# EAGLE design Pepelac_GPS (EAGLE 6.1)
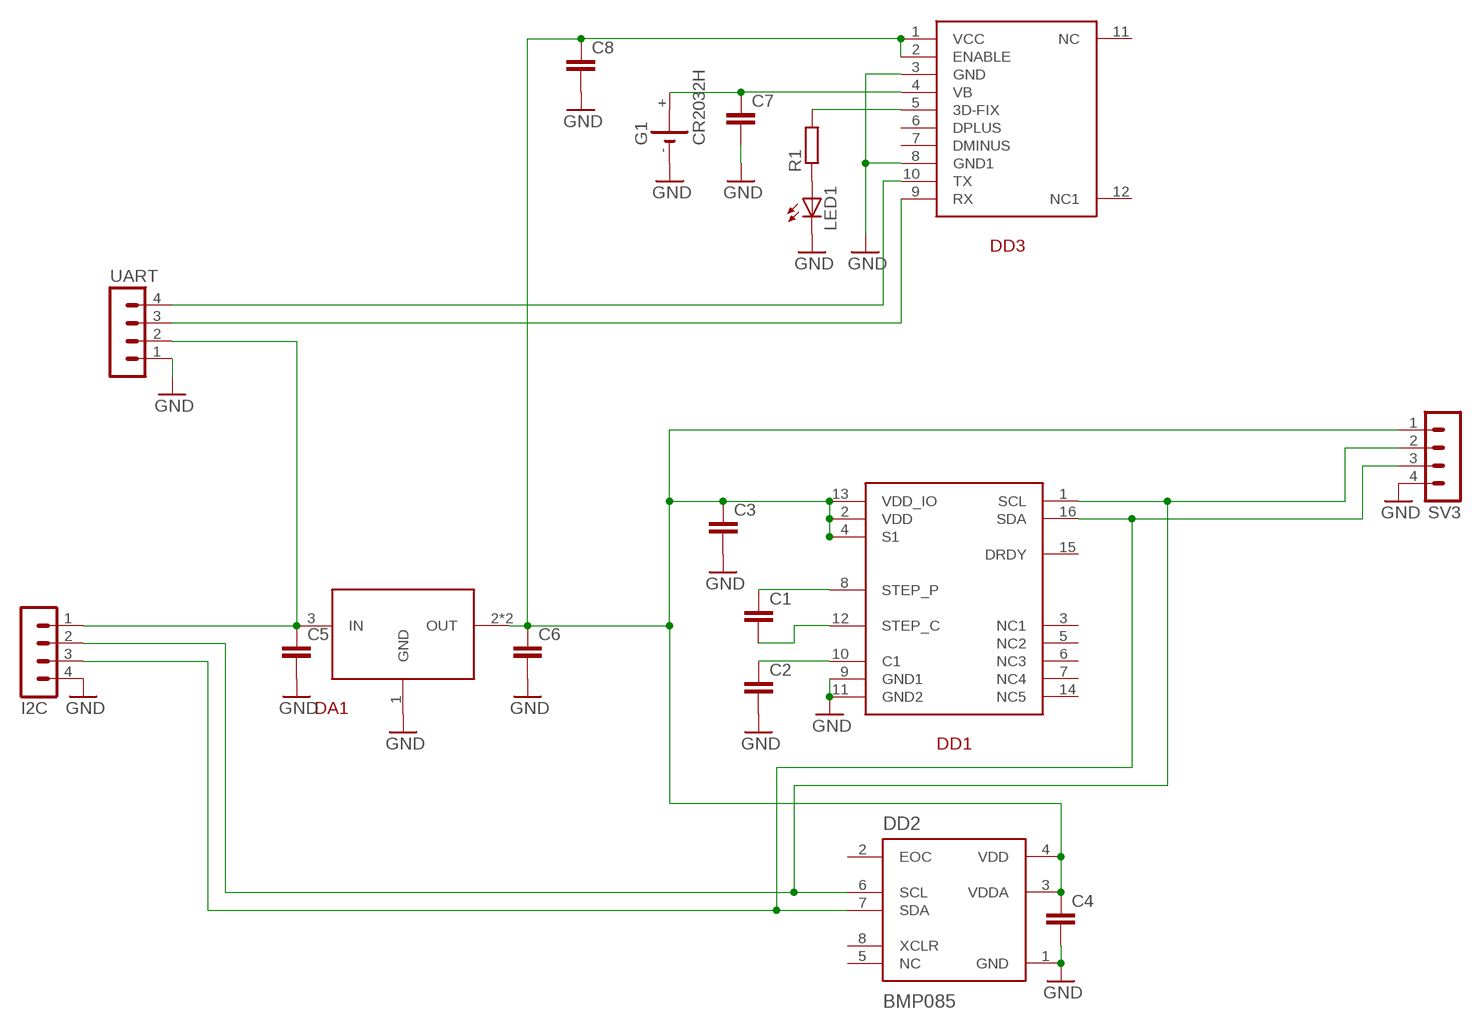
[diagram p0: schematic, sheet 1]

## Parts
C1  C-EUC3216  [C3216]
C2  C-EUC3216  [C3216]
C3  C-EUC3216  [C3216]
C4  C-EUC3216  [C3216]
C5  C-EUC3216  [C3216]
C6  C-EUC3216  [C3216]
C7  C-EUC3216  [C3216]
C8  C-EUC3216  [C3216]
DA1  1117  [SOT223-W]
DD1  HMC5883L  [LCC-16]
DD2  BMP085  [QFN127P500X500X120-8N]
DD3  FGPMMOPA6B  [FGPMMOPA6B]
G1  CR2032H  [CR2032H]
I2C  MA04-1  [MA04-1]
LED1  LEDKA-3528ASYC  [KA-3528ASYC]
R1  R-EU_M3216  [M3216]
SV3  MA04-1  [MA04-1]
UART  MA04-1  [MA04-1]

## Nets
GND: C2.2 C3.2 C4.2 C5.2 C6.2 C7.2 C8.2 DA1.1(GND) DD1.9(GND1) DD1.11(GND2) DD2.1(GND) DD3.3(GND) DD3.8(GND1) G1.- I2C.4 LED1.C SV3.4 UART.1
N$2: C5.1 DA1.3(IN) I2C.1 UART.2
N$3: C3.1 C4.1 C6.1 C8.1 DA1.2(OUT) DA1.4(OUT) DD1.2(VDD) DD1.4(S1) DD1.13(VDD_IO) DD2.3(VDDA) DD2.4(VDD) DD3.1(VCC) DD3.2(ENABLE) SV3.1
N$4: LED1.A R1.1
N$5: DD1.16(SDA) DD2.7(SDA) I2C.3 SV3.3
N$6: DD1.1(SCL) DD2.6(SCL) I2C.2 SV3.2
N$8: C7.1 DD3.4(VB) G1.+
N$11: DD3.5(3D-FIX) R1.2
N$15: DD3.10(TX) UART.4
N$16: DD3.9(RX) UART.3
N$17: C1.1 DD1.8(STEP_P)
N$18: C1.2 DD1.12(STEP_C)
N$19: C2.1 DD1.10(C1)
Unconnected: DD1.3(NC1) DD1.5(NC2) DD1.6(NC3) DD1.7(NC4) DD1.14(NC5) DD1.15(DRDY) DD2.2(EOC) DD2.5(NC) DD2.8(XCLR) DD3.6(DPLUS) DD3.7(DMINUS) DD3.11(NC) DD3.12(NC1) G1.+@1(+)

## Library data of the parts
C1-C8 = resistor:C-EU: CAPACITOR, European symbol
DA1 = pepelac:1117
DD1 = pepelac:HMC5883L
DD2 = pepelac:BMP085: BMP085 Digital pressure sensor
DD3 = pepelac:FGPMMOPA6B
G1 = battery:CR2032H: LI BATTERY Varta
I2C SV3 UART = con-lstb:MA04-1: PIN HEADER; OC_FARNELL: unknown; OC_NEWARK: unknown
LED1 = led:LED: LED
R1 = resistor:R-EU_: RESISTOR, European symbol

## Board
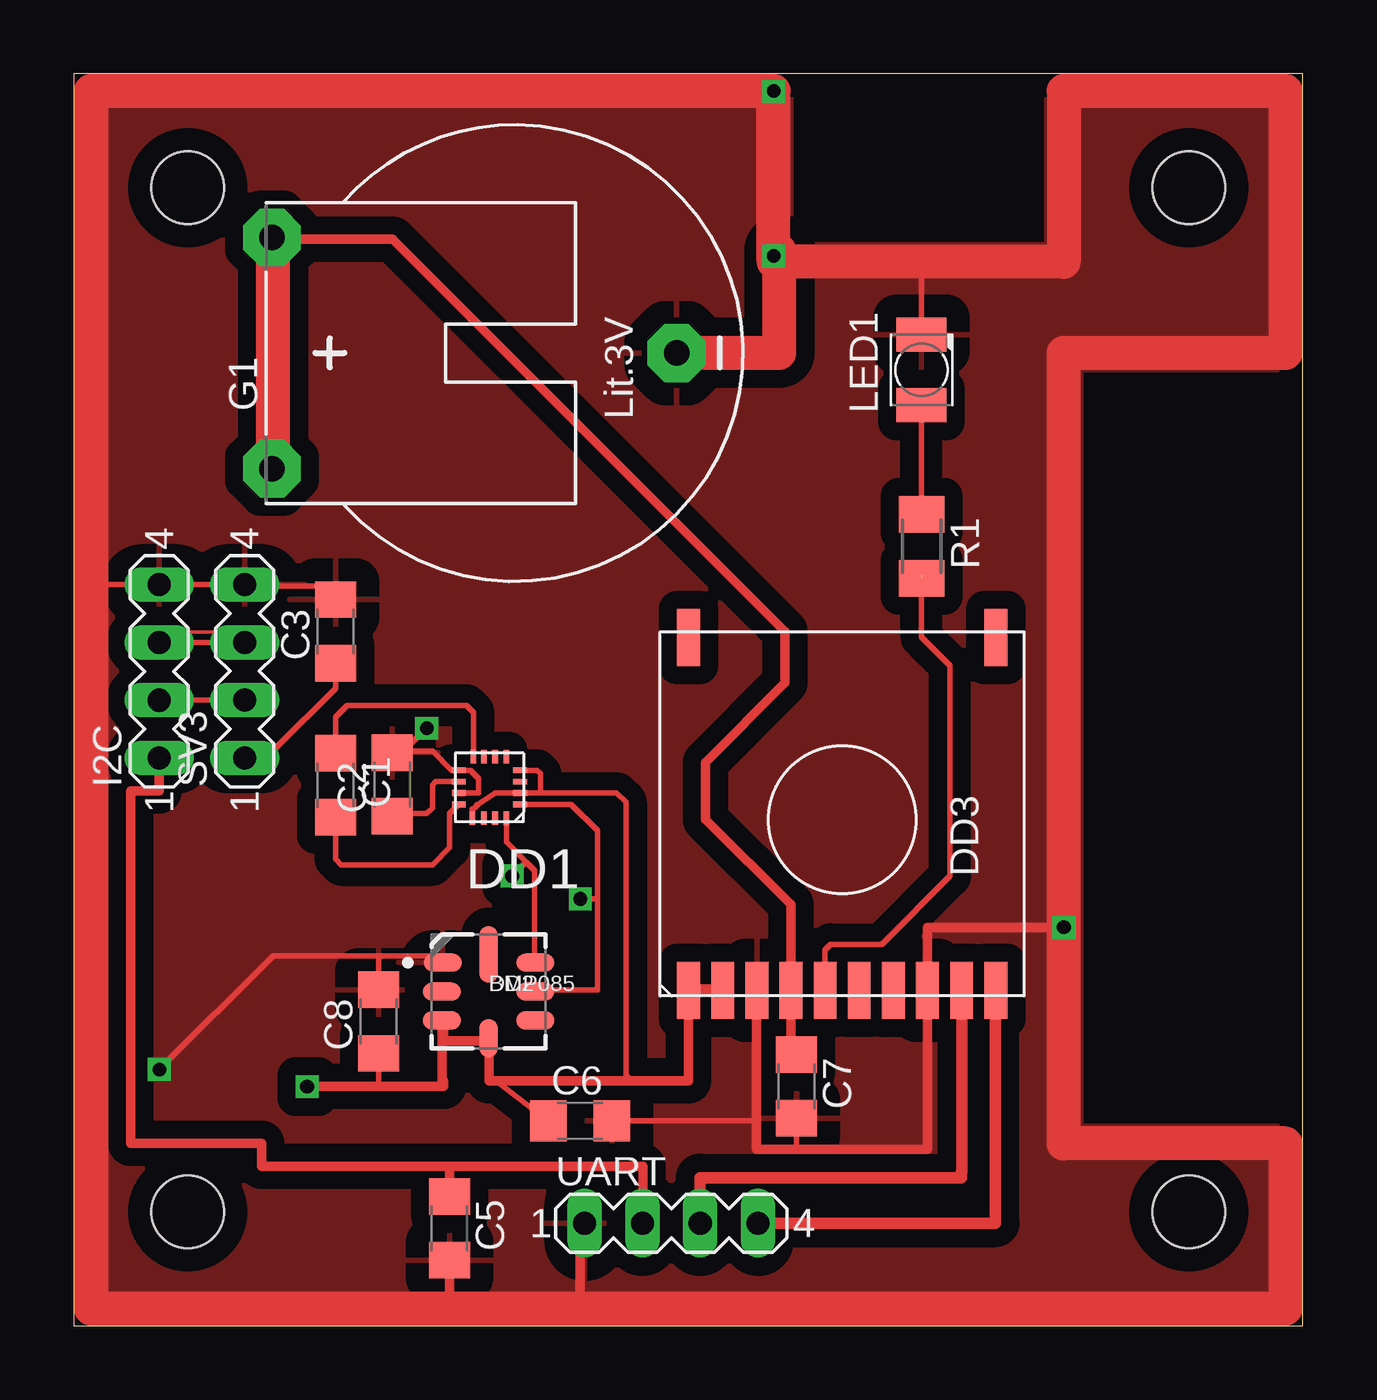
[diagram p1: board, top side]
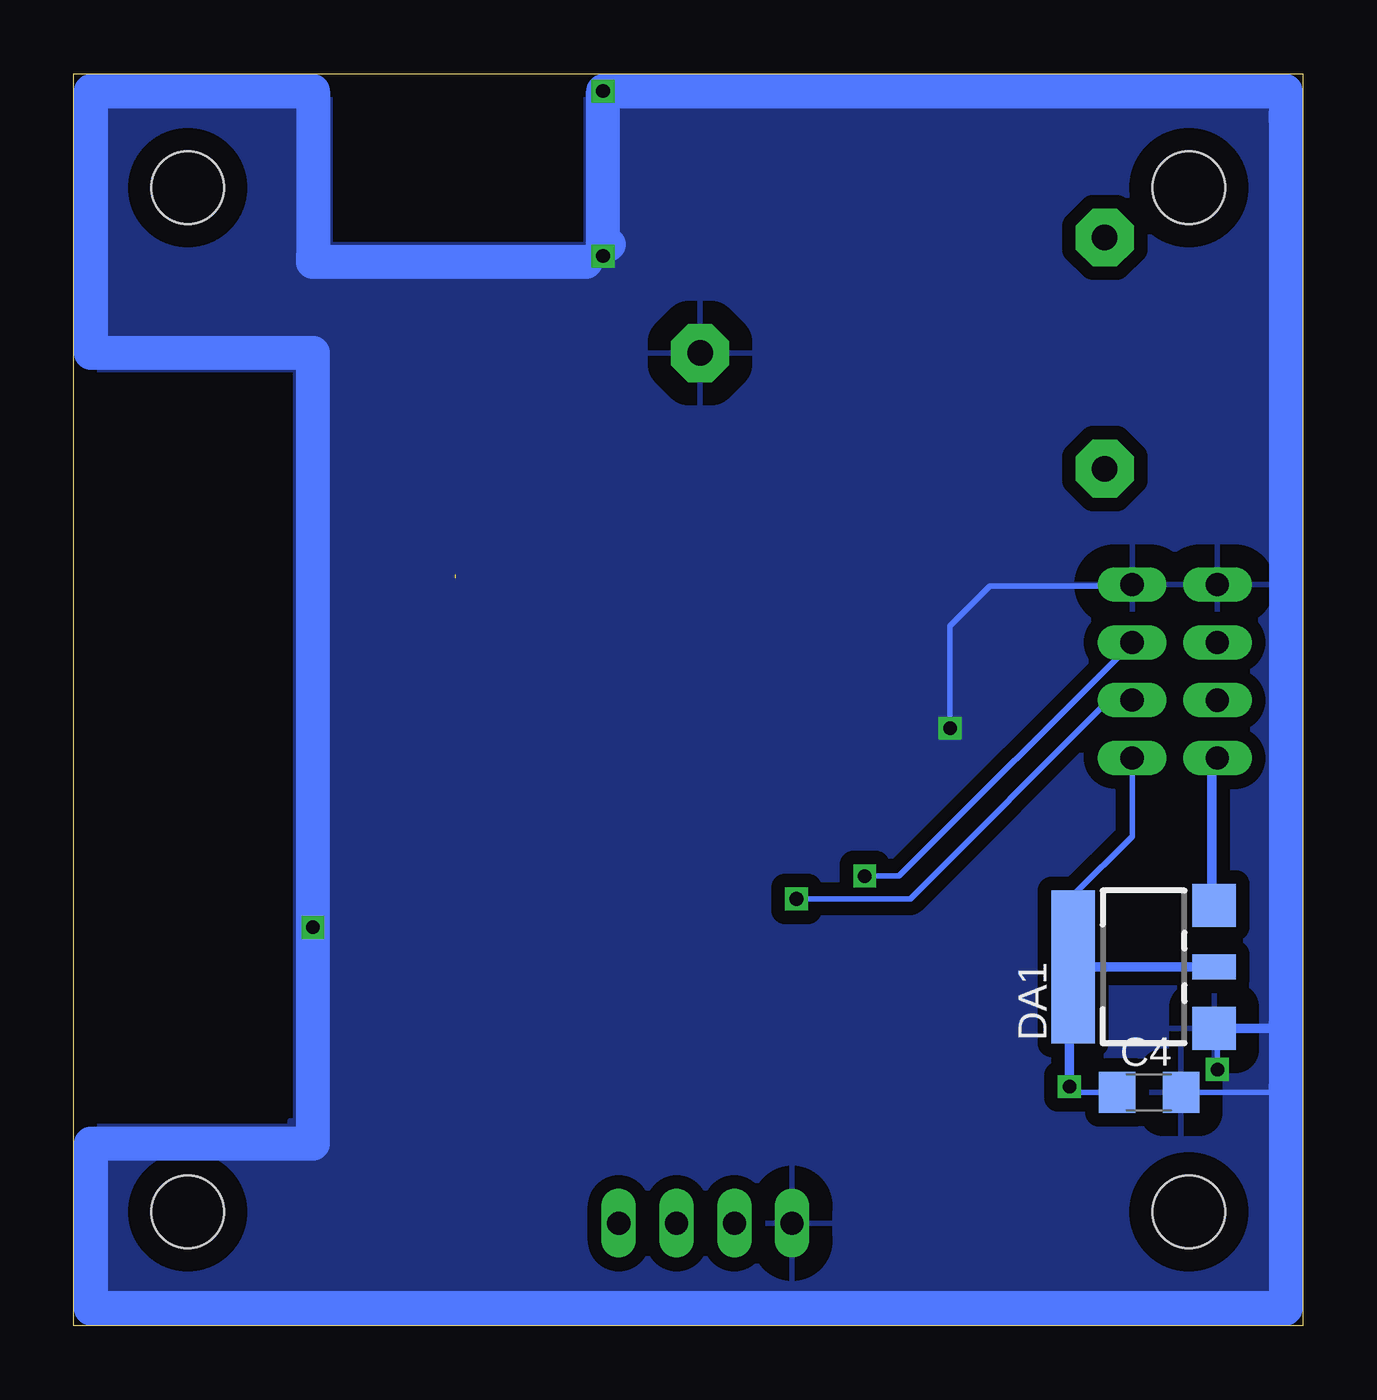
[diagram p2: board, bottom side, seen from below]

Size 54 x 55 mm. Coordinates in mm from the lower left corner, seen from the top.
Outline: 0,0 54,0 54,55 0,55 0,0
Copper layers (1*16): Top 0.035mm / dielectric 1.5mm / Bottom 0.035mm
Design rules: minimum track width 6mil, minimum drill 30mil, track to track 6mil, track to pad 6mil, pad to pad 8mil, via to via 8mil, smd to smd 8mil, copper to edge 40mil, drill to drill 8mil, minimum pad ring 10mil, minimum via ring 8mil, stop-mask expansion 4mil, vias tented up to drill 0mil, thermal gap 40mil
Holes 3.2 mm at 5,50 49,50 49,5 5,5

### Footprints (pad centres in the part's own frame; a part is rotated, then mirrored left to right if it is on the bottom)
C3216 = smd 1.6 x 1.8: 1 -1.4,0; 2 1.4,0
SOT223-W = smd 1.9 x 1.9: 1 -2.7,-3.1; 3 2.7,-3.1 | smd 1.1 x 1.9: 2 0,-3.1 | smd 6.7 x 1.9: 4 0,3.1
LCC-16 = smd 0.6 x 0.25: 1 -1.35,0.85; 2 -1.35,0.35; 3 -1.35,-0.15; 4 -1.35,-0.65; 9 1.35,-0.65; 10 1.35,-0.15; 11 1.35,0.35; 12 1.35,0.85 | smd 0.25 x 0.6: 5 -0.75,-1.25; 6 -0.25,-1.25; 7 0.25,-1.25; 8 0.7,-1.25; 13 0.75,1.45; 14 0.25,1.45; 15 -0.25,1.45; 16 -0.75,1.45
QFN127P500X500X120-8N = smd 1.67 x 0.8: 1 -2.01,1.27; 2 -2.05,0; 3 -2.05,-1.27; 5 2.05,-1.27; 6 2.05,0; 7 2.05,1.27 | smd 0.8 x 1.67: 4 0,-2.05 | smd 0.8 x 2.5: 8 0,1.63
FGPMMOPA6B = smd 2.5 x 1: 1 -7.5,6.75; 2 -7.5,5.25; 3 -7.5,3.75; 4 -7.5,2.25; 5 -7.5,0.75; 6 -7.5,-0.75; 7 -7.5,-2.25; 8 -7.5,-3.75; 9 -7.5,-5.25; 10 -7.5,-6.75; 11 8,6.75; 12 8,-6.75
CR2032H = drill 1.118 pad 2.54 octagon: + 5.08,10.795; +@1 -5.08,10.795; - 0,-6.985
MA04-1 = drill 1.016 long: 1 -3.81,0; 2 -1.27,0; 3 1.27,0; 4 3.81,0
KA-3528ASYC = smd 1.5 x 2.2: A -1.55,0; C 1.55,0
M3216 = smd 1.6 x 2: 1 -1.4,0; 2 1.4,0

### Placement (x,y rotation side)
C1  11.49,23.74 270 top
C2  13.99,23.78 90 top
C3  11.5,30.51 90 top
C4  6.76,10.25 0 bottom
C5  16.5,4.27 270 top
C6  22.24,9 0 top
C7  31.75,10.51 270 top
C8  13.39,13.36 90 top
DA1  7,15.76 90 bottom
DD1  18.26,23.75 180 top
DD2  18.22,14.68 0 top
DD3  33.76,22.23 90 top
G1  19.5,42.73 90 top
I2C  3.75,28.75 90 top
LED1  37.25,41.99 90 top
R1  37.25,34.24 270 top
SV3  7.5,28.75 90 top
UART  26.25,4.5 0 top

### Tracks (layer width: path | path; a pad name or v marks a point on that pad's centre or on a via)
GND  (via drill 0.6)
  Top 0.25: SV3.4 I2C.4 | SV3.4 0.94,32.56 0.75,32.75 | G1.- 30.48,42.73 31.25,43.5 31.25,46.5 v30.75,47 | DD1.11 17.79,23.4 17.79,24.03 17.46,24.36 17.46,24.37 17.43,24.4 DD1.9 16.6,24.4 15.75,25.25 14.06,25.25 C2.2 14.43,25.18 v15.5,26.25 | C3.2 11.35,31.91 10.75,32.5 7.56,32.5 SV3.4 | C6.2 30,9 | 30,9 | C7.2 31.75,7.75 | LED1.C 37.25,46.75 | C8.2 13.39,16.14 13.5,16.25 | 13.5,16.25 15.91,16.25 DD2.1 | 13.5,16.25 8.75,16.25 v3.75,11.25
  Top 0.406: DD3.3 30,9 30,7.75 31.75,7.75 37.5,7.75 37.5,14.75 | DD3.8 37.5,17.5 v43.5,17.5 | 22.46,4.5 22.25,4.5 22.25,0.75 | C5.2 16.5,1 16.75,0.75
  Top 0.5: UART.1 22.46,4.5 | DD3.3 | DD3.8
  Top 1.5: 0.75,54.25 0.75,32.75 0.75,0.75 16.75,0.75 22.25,0.75 53.25,0.75 53.25,8 43.5,8 v43.5,17.5 43.5,42.75 53.25,42.75 53.25,54.25 43.5,54.25 43.5,46.75 37.25,46.75 30.75,46.75 v30.75,47 v30.75,54.25 0.75,54.25
  Bottom 0.25: C4.2 1,10.25 0.75,10.5 | v15.5,26.25 15.5,30.75 13.75,32.5 7.56,32.5 SV3.4 | v3.75,11.25 3.75,12.91 DA1.1
  Bottom 0.406: DA1.1 0.94,13.06 0.75,13.25
  Bottom 0.5: 43.5,47 31.5,47 31.5,46.75
  Bottom 1.5: 31.5,46.75 43.5,46.75 43.5,47 43.5,54.25 53.25,54.25 53.25,42.75 43.5,42.75 v43.5,17.5 43.5,8 53.25,8 53.25,0.75 0.75,0.75 0.75,10.5 0.75,13.25 0.75,53 | 30.5,47.5 30.75,47.5 v30.75,54.25 0.75,54.25 0.75,53.25
  pour Bottom (isolate 0.6): 0,0 54,0 54,8.75 44.5,8.75 44.5,9 44.25,9 44.25,42 54,42 54,55 42.75,55 42.75,47.5 31.5,47.5 31.5,55 0,55
  pour Top (isolate 0.8): 0,55 31.5,55 31.5,47.5 42.75,47.5 42.75,47.75 42.75,55 54,55 54,42 44.25,42 44.25,8.75 54,8.75 54,0 0,0
N$1
  Top 1.5: 26.5,42.75 31,42.75 31,47.25
N$2
  Top 0.406: UART.2 25,4.5 25,7 16.5,7 | 16.5,7 8.25,7 8.25,8 2.5,8 2.5,23.5 3.75,23.5 I2C.1 | C5.1 16.5,7
  Bottom 0.406: I2C.1 4,24.94 4,18.5 3.9,18.5 DA1.3
N$3  (via drill 0.6)
  Top 0.152: 8.89,25.39 8.89,25.4 7.62,25.4 SV3.1
  Top 0.25: 20.5,23.4 DD1.2 19.51,23.4 19.5,23.41 | 20.5,23.4 23.85,23.4 24.25,23 24.25,11 24.5,10.75 | C6.1 18.66,10.66 18.75,10.75 | C3.1 11.5,28 8.89,25.39 8.75,25.25 7.75,25.25 7.5,25 | DD1.13 17.51,22.71 17.55,22.71 17.69,22.85 | 17.69,22.85 | 17.69,22.85 17.73,22.89 17.63,22.77 17.75,22.89 18.5,23.4 18.52,23.41 19.5,23.41 | 19.5,23.41 19.6,23.41 DD1.2 | DD1.4 20.35,24.4 20.5,24.25 20.5,23.4 | C8.1 13.39,10.61 13.5,10.5
  Top 0.406: v10.25,10.5 13.5,10.5 16.25,10.5 16.25,10.75 16.17,10.75 DD2.3 16.25,13.41 16.25,12.5 18.22,12.5 DD2.4 18.25,12.63 18.25,10.75 18.75,10.75 24.5,10.75 27,10.75 27,11 27.01,11 DD3.1
  Top 0.5: 27.01,15 DD3.1 27,14.75 28.51,14.75 DD3.2
  Bottom 0.25: DA1.4 10.1,18.91 7.5,21.5 SV3.1 | SV3.1 | C4.1 10,10.25 v10.25,10.5
  Bottom 0.406: DA1.2 DA1.4 10.25,15.76 v10.25,10.5
N$4
  Top 0.25: R1.1 LED1.A
N$5  (via drill 0.6)
  Top 0.152: I2C.3 3.81,30.48 6.35,30.48 SV3.3
  Top 0.25: DD1.16 19.01,21.24 19.88,20.38 | 19.88,20.38 20.25,20 20.25,15.97 DD2.7 | v19.25,19.75 19.88,20.38 | SV3.3 3.77,30.02 3.75,30
  Bottom 0.25: SV3.3 7.5,30 17.75,19.75 v19.25,19.75
N$6  (via drill 0.6)
  Top 0.25: DD1.1 21.85,22.9 23,21.75 23,18.75 | 23,18.75 23,14.75 20.34,14.75 DD2.6 | v22.25,18.75 23,18.75 | SV3.2 I2C.2
  Bottom 0.25: SV3.2 8.52,27.48 17.25,18.75 v22.25,18.75
N$8
  Top 0.406: C7.1 31.5,11.91 DD3.4 31.5,18.5 27.75,22.25 27.75,24.75 31.25,28.25 31.25,30.5 14,47.75 9.25,47.75 8.77,47.75 G1.+
  Top 0.5: DD3.4
  Top 1.5: 8.75,38 8.75,47.75 9.25,47.75
N$11  (1 unrouted)
  Top 0.152: 36.83,33.02 R1.2 | 33.02,16.51 33.01,16.51
  Top 0.25: DD3.5 33.01,16.51 33.25,16.75 35.5,16.75 38.5,19.75 38.5,29 37.25,30.25 37.25,33
N$15
  Top 0.5: UART.4 40.5,4.5 DD3.10 | DD3.10 | DD3.10 40.5,14.75
N$16
  Top 0.5: UART.3 27.5,4.5 27.5,6.5 39,6.5 39,6.75 39.01,6.75 DD3.9
N$17
  Top 0.152: C1.1 11.43,25.4 11.5,25.4
  Top 0.25: DD1.8 17.56,26.94 17.25,27.25 12,27.25 11.5,26.75 11.5,25.4 11.5,25.25
N$18
  Top 0.25: C1.2 11.49,20.51 11.75,20.25 15.75,20.25 16.5,21 16.5,22.5 DD1.12
N$19
  Top 0.25: DD1.10 15.9,23.9 15.75,23.75 15.75,22.75 15.5,22.5 14.11,22.5 C2.1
